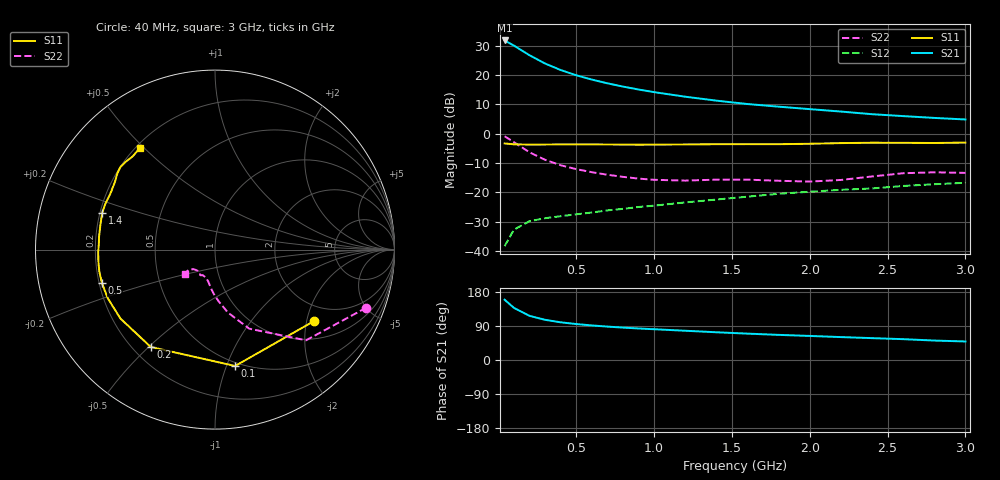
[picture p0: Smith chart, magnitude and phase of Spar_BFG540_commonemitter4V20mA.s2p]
! Filename:  BFG540C.S2P  Version:  3.0
! NXP part #: BFG540  Date: Feb 1992
! Bias condition: Vce=4V, Ic=20mA
! IN LINE PINNING: same data as with cross emitter pinning.
#  MHz  S  MA  R  50
! Freq  S11  S21  S12  S22  !GUM [dB]
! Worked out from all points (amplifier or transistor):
!   21 points, 40 MHz to 3 GHz, reference 50 ohm
!   highest |S21| = 31.8 dB at 40 MHz (marker M1)
!   |S21| within 3 dB of that: start of sweep to 137.6 MHz
!   unconditionally stable (mu >= 1): 905.7 MHz to end of sweep
!   at 300 MHz: K = 0.50, MSG = 26.4 dB, |S12| = -28.9 dB
!   at 1 GHz: K = 1.05, MAG = 18.0 dB, |S12| = -24.6 dB
!   at 3 GHz: K = 1.17, MAG = 8.3 dB, |S12| = -16.8 dB
!   lowest NFmin = 1.50 dB at 900 MHz
!   S11 on the Smith chart (normalised r, x): 40 MHz: 1.49, -2.21; 100 MHz: 0.47, -1.07; 200 MHz: 0.27, -0.51; 500 MHz: 0.21, -0.14; 1.4 GHz: 0.21, +0.15; 3 GHz: 0.22, +0.49
40  0.68 -35.9  39.02 159.1  0.012 73.1  0.903 -21.0
100  0.658 -80.2  31.86 137.5  0.023 56.1  0.716 -44.9
200  0.65 -123.4  21.8 116.5  0.032 44.4  0.48 -66.6
300  0.652 -143.9  15.76 106.0  0.036 41.8  0.358 -78.4
400  0.656 -155.6  12.2 99.5  0.039 42.9  0.289 -86.0
500  0.657 -163.5  9.939 94.9  0.042 44.6  0.248 -91.4
600  0.656 -169.4  8.383 91.2  0.045 47.4  0.22 -95.4
700  0.653 -174.4  7.24 88.2  0.049 49.2  0.199 -98.6
800  0.651 -178.7  6.368 85.5  0.052 51.2  0.183 -101.7
900  0.648 177.4  5.675 83.2  0.056 53.4  0.171 -105.2
1000  0.65 173.6  5.117 81.2  0.059 55.2  0.163 -108.8
1200  0.654 167.1  4.276 77.2  0.067 57.7  0.158 -115.6
1400  0.661 162.0  3.664 73.2  0.075 59.1  0.164 -119.4
1600  0.662 157.2  3.206 69.6  0.084 61.6  0.164 -120.4
1800  0.661 151.9  2.891 66.3  0.094 61.9  0.157 -122.3
2000  0.672 146.3  2.623 63.5  0.102 63.2  0.152 -129.0
2200  0.69 142.0  2.385 60.5  0.11 63.4  0.162 -137.9
2400  0.7 138.9  2.149 57.7  0.116 64.5  0.186 -142.5
2600  0.698 135.7  1.994 55.0  0.128 63.8  0.211 -141.9
2800  0.693 131.4  1.857 51.3  0.137 61.9  0.219 -140.0
3000  0.704 126.3  1.747 48.9  0.145 62.8  0.214 -141.5
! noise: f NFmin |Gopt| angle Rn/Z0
900  1.5  0.281  159  0.11
2000  2.2  0.518  -157  0.12
